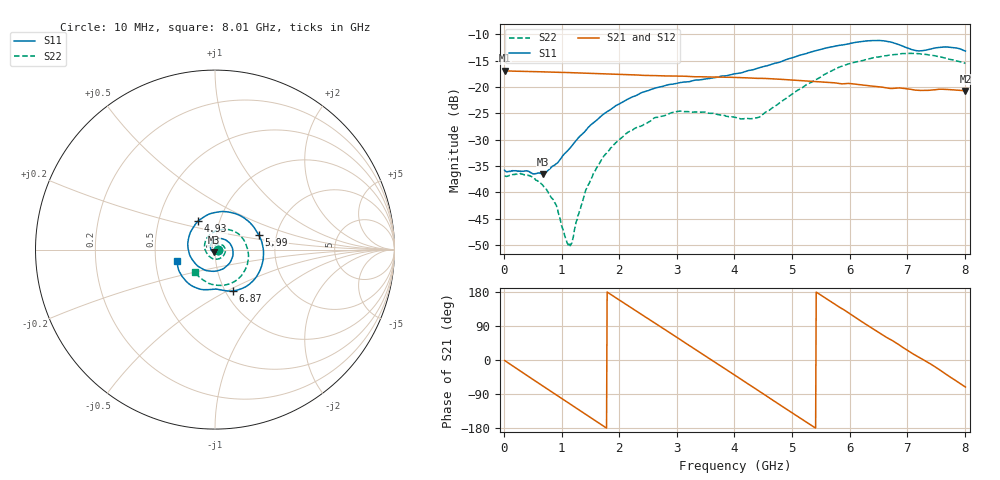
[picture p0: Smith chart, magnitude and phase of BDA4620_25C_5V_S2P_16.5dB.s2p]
!Agilent Technologies,E5071B,MY42404982,A.09.10
!Date: Wed May 06 09:01:45 2026
!Data & Calibration Information:
!Freq	S11:SOLT2(ON)	S21:SOLT2(ON)	S12:SOLT2(ON)	S22:SOLT2(ON)
# Hz S RI R 50
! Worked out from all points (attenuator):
!   801 points, 10 MHz to 8.01 GHz, reference 50 ohm
!   highest |S21| = -16.92 dB at 10 MHz (marker M1); lowest = -20.7 dB at 8.01 GHz (marker M2)
!   lowest |S11| = -36.6 dB at 680 MHz (marker M3), VSWR 1.03, Z = 49.5 - j1.41 ohm
!   |S11| at or under -10 dB: start of sweep to end of sweep
!   |S22| runs from -50.2 to -13.6 dB; largest |S21 - S12| = 0.00065
!   S11 on the Smith chart (normalised r, x): 10 MHz: 1.03, -0.00; 4.93 GHz: 0.79, +0.26; 5.99 GHz: 1.62, +0.28; 6.87 GHz: 1.08, -0.53; 8.01 GHz: 0.65, -0.08
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1e7  0.0162 -0.00114  0.1425 -0.00304  0.1427 -0.0031  0.0142 -0.000507
4.2e8  0.00837 -0.0134  0.1025 -0.0957  0.1026 -0.096  0.0134 -0.00544
6.8e8  -0.00436 -0.0142  0.049 -0.1302  0.049 -0.1304  0.00876 -0.0075
8.9e8  -0.0162 -0.00883  -0.00131 -0.138  -0.00147 -0.1384  0.00323 -0.00718
1.13e9  -0.0249 0.00674  -0.0573 -0.1243  -0.0575 -0.1245  -0.00259 -0.0018
1.19e9  -0.0257 0.0118  -0.0698 -0.1172  -0.07 -0.1175  -0.00353 0.000263
1.35e9  -0.0247 0.0254  -0.099 -0.0929  -0.099 -0.0929  -0.00522 0.00575
1.58e9  -0.0137 0.045  -0.126 -0.0465  -0.1262 -0.0465  -0.00417 0.0154
1.87e9  0.0149 0.0605  -0.1311 0.0201  -0.1314 0.0201  0.00448 0.0265
2.68e9  0.0995 -0.00204  -0.00295 0.1279  -0.00285 0.1281  0.0483 0.0188
3.41e9  0.031 -0.1127  0.1181 0.0414  0.1183 0.0414  0.0443 -0.0372
4.01e9  -0.1012 -0.0869  0.0938 -0.0798  0.0938 -0.0801  -0.0153 -0.0493
4.42e9  -0.151 0.0141  0.0185 -0.1194  0.0183 -0.1196  -0.0503 -0.0118
4.93e9  -0.0945 0.1584  -0.0788 -0.0867  -0.079 -0.0868  -0.0415 0.0689
5.35e9  0.0429 0.2123  -0.1126 -0.012  -0.1127 -0.012  0.0251 0.109
5.99e9  0.2439 0.0804  -0.0594 0.0901  -0.0596 0.0902  0.1534 0.0642
6.34e9  0.2649 -0.0724  0.00233 0.1027  0.00241 0.1028  0.1847 -0.0125
6.68e9  0.1754 -0.2043  0.0538 0.0808  0.054 0.081  0.1743 -0.0984
6.87e9  0.0978 -0.2302  0.0763 0.0614  0.0765 0.0614  0.1497 -0.1414
7.19e9  0.00649 -0.2199  0.0918 0.0136  0.0921 0.0139  0.0762 -0.193
7.55e9  -0.1005 -0.2147  0.0865 -0.0397  0.0866 -0.0396  -0.0195 -0.193
8.01e9  -0.21 -0.062  0.0294 -0.0869  0.0296 -0.0872  -0.1118 -0.1242
